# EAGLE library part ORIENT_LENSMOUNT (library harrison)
Orient chip
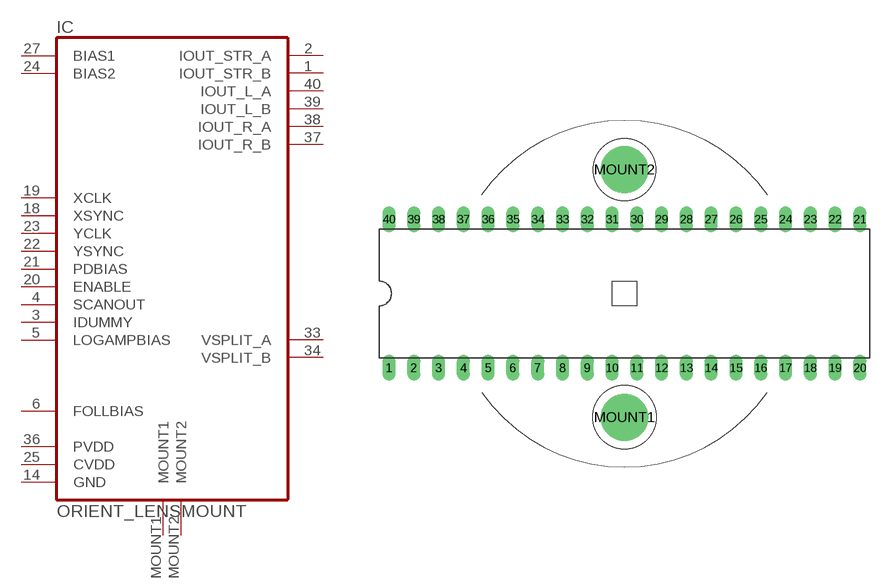
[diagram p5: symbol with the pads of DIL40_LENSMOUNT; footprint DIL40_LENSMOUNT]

Designator prefix IC

## ORIENT_LENSMOUNT  [DIL40_LENSMOUNT]
1  IOUT_STR_B  pas
2  IOUT_STR_A  pas
3  IDUMMY  pas
4  SCANOUT  out
5  LOGAMPBIAS  pas
6  FOLLBIAS  in
14  GND  pwr
18  XSYNC  out
19  XCLK  in
20  ENABLE  in
21  PDBIAS  in
22  YSYNC  out
23  YCLK  in
24  BIAS2  pas
25  CVDD  pwr
27  BIAS1  pas
33  VSPLIT_A  in
34  VSPLIT_B  in
36  PVDD  pwr
37  IOUT_R_B  pas
38  IOUT_R_A  pas
39  IOUT_L_B  pas
40  IOUT_L_A  pas
MOUNT1  MOUNT1  pas
MOUNT2  MOUNT2  pas

## Footprint DIL40_LENSMOUNT (pad centres in mm)
drill 0.813 long: 1 -24.13,-7.62; 2 -21.59,-7.62; 3 -19.05,-7.62; 4 -16.51,-7.62; 5 -13.97,-7.62; 6 -11.43,-7.62; 7 -8.89,-7.62; 8 -6.35,-7.62; 9 -3.81,-7.62; 10 -1.27,-7.62; 11 1.27,-7.62; 12 3.81,-7.62; 13 6.35,-7.62; 14 8.89,-7.62; 15 11.43,-7.62; 16 13.97,-7.62; 17 16.51,-7.62; 18 19.05,-7.62; 19 21.59,-7.62; 20 24.13,-7.62; 21 24.13,7.62; 22 21.59,7.62; 23 19.05,7.62; 24 16.51,7.62; 25 13.97,7.62; 26 11.43,7.62; 27 8.89,7.62; 28 6.35,7.62; 29 3.81,7.62; 30 1.27,7.62; 31 -1.27,7.62; 32 -3.81,7.62; 33 -6.35,7.62; 34 -8.89,7.62; 35 -11.43,7.62; 36 -13.97,7.62; 37 -16.51,7.62; 38 -19.05,7.62; 39 -21.59,7.62; 40 -24.13,7.62
drill 3.81: MOUNT1 0,-12.7; MOUNT2 0,12.7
